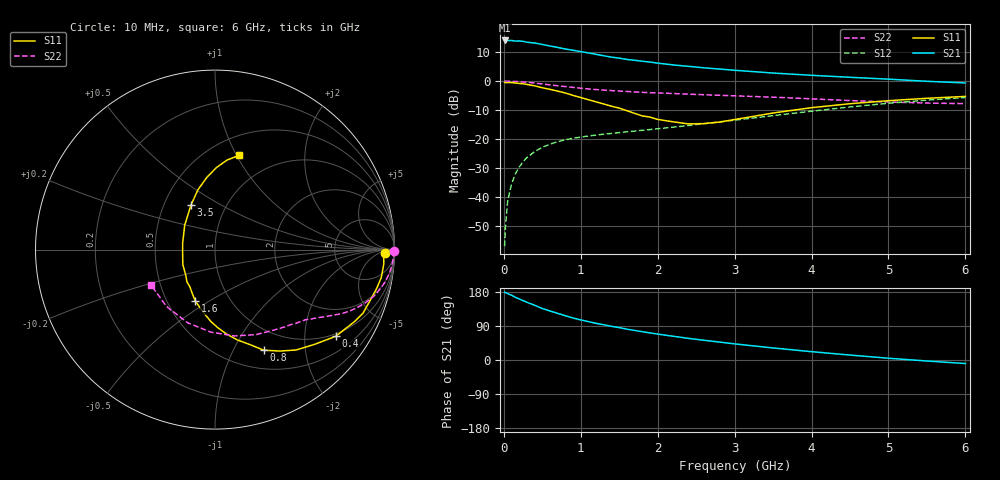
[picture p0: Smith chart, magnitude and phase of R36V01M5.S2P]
! SIEMENS Small Signal Semiconductors
! BFR181
! Si NPN RF Bipolar Junction Transistor in SOT23
! VCE = 6 V  IC = 1.5 mA
! Common Emitter S-Parameters:  May  1996
# GHz  S  MA  R  50
!  f  S11  S21  S12  S22
! GHz  MAG  ANG  MAG  ANG  MAG  ANG  MAG  ANG
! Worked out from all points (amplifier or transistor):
!   36 points, 10 MHz to 6 GHz, reference 50 ohm
!   highest |S21| = 14.0 dB at 10 MHz (marker M1)
!   |S21| within 3 dB of that: start of sweep to 808.8 MHz
!   unconditionally stable (mu >= 1): 1.796 GHz to 3.528 GHz
!   at 250 MHz: K = 0.20, MSG = 20.8 dB, |S12| = -27.9 dB
!   at 1.4 GHz: K = 0.87, MSG = 13.2 dB, |S12| = -18.1 dB
!   at 6 GHz: K = 0.86, MSG = 2.5 dB, |S12| = -5.7 dB
!   S11 on the Smith chart (normalised r, x): 10 MHz: 33, -11; 400 MHz: 0.92, -2.84; 800 MHz: 0.72, -1.33; 1.6 GHz: 0.69, -0.44; 3.5 GHz: 0.68, +0.37; 6 GHz: 0.69, +1.03
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0.01  0.947 -1.0  5.034 179.1  0.0014 95.0  0.9979 -0.5
0.02  0.9398 -1.9  4.916 177.8  0.0029 85.2  0.9983 -1.0
0.05  0.944 -4.8  5.02 175.3  0.0085 86.8  0.9949 -2.2
0.1  0.9395 -9.5  5.03 171.0  0.0166 85.0  0.9912 -4.4
0.15  0.9259 -13.7  4.913 165.5  0.0249 81.3  0.9847 -6.7
0.2  0.9083 -18.6  4.927 161.1  0.0326 78.6  0.9749 -8.7
0.25  0.8978 -23.2  4.859 156.6  0.0404 75.0  0.9644 -10.8
0.4  0.828 -35.7  4.545 144.5  0.0604 68.7  0.9252 -16.1
0.5  0.765 -43.7  4.291 135.8  0.0715 64.5  0.891 -19.3
0.7  0.6704 -57.5  3.815 123.0  0.0893 58.3  0.8302 -24.1
0.8  0.6223 -64.2  3.58 116.8  0.0968 55.6  0.8031 -26.0
0.9  0.5648 -69.7  3.401 110.8  0.1028 53.9  0.7772 -27.6
1.1  0.4754 -82.1  3.066 101.2  0.1125 51.6  0.7321 -30.4
1.3  0.4012 -93.3  2.736 92.9  0.121 50.3  0.6978 -32.7
1.6  0.3077 -110.8  2.364 81.4  0.1327 49.7  0.6613 -35.8
1.9  0.2382 -131.0  2.132 71.5  0.1452 51.0  0.6299 -38.9
2.2  0.1977 -155.1  1.901 62.7  0.1597 51.8  0.6095 -42.5
2.8  0.195 153.3  1.615 47.4  0.1967 53.6  0.5682 -50.6
3.5  0.2807 118.6  1.376 31.8  0.2526 52.7  0.5264 -64.1
4.5  0.406 96.3  1.162 13.0  0.3571 46.1  0.4601 -93.0
5.5  0.5038 82.3  0.991 -2.7  0.4686 34.1  0.4164 -130.4
6  0.5428 75.5  0.928 -9.3  0.5204 26.5  0.4071 -150.7
